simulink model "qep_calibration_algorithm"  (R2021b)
settings: Solver=FixedStepDiscrete  StartTime=0.0  StopTime=10.0  RelTol=1e-3
InitFcn:
  | qep_calibration_data;
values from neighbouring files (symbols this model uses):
  PWM_frequency = 20e3    (= 20000)    [qep_calibration_data.m]    (also in foc_qep_data.m; open_loop_data.m)
  Ts = 1/PWM_frequency    (= 5e-05)    [qep_calibration_data.m]    (also in foc_qep_data.m; open_loop_data.m)
undefined symbols (not defined in the file or in its folder): bits, motor
libraries: mcbcontrolslib x4, simulink x2, mcbpositiondecoderlib x2

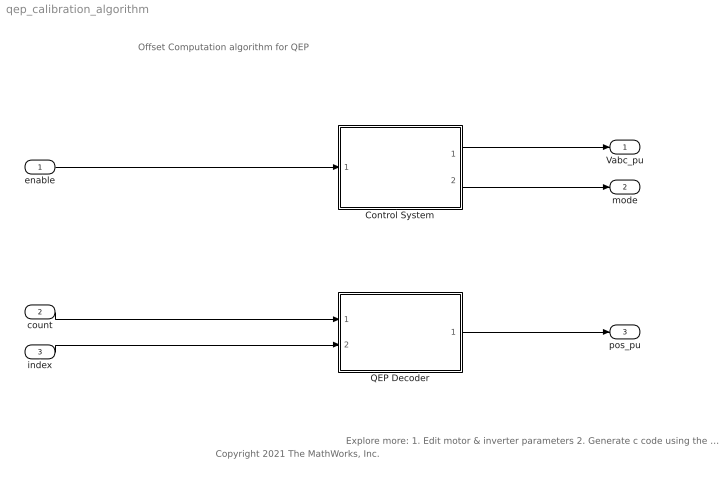
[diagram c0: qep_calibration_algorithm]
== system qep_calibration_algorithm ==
  note: Offset Computation algorithm for QEP
  note: Explore more: 1. Edit motor & inverter parameters 2. Generate c code using the 'Embedded Coder' app 3. Integrate generated code with driver code 4. Control motor via host model
  note: Copyright 2021 The MathWorks, Inc.
  enable : Inport  OutDataTypeStr=boolean
  count : Inport  Port=2  OutDataTypeStr=uint16
  index : Inport  Port=3  OutDataTypeStr=uint16
  Control System : Subsystem
  QEP Decoder : Subsystem
  Vabc_pu : Outport  OutDataTypeStr=dataType  VectorParamsAs1DForOutWhenUnconnected=off
  mode : Outport  Port=2  OutDataTypeStr=dataType
  pos_pu : Outport  Port=3  OutDataTypeStr=dataType
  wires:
  enable/1 -> Control System/1(Enable)
  Control System/1(Vabc_pu) -> Vabc_pu/1
  Control System/2(mode) -> mode/1
  count/1 -> QEP Decoder/1(Count)
  index/1 -> QEP Decoder/2(IndexCount)
  QEP Decoder/1(ϴe) -> pos_pu/1

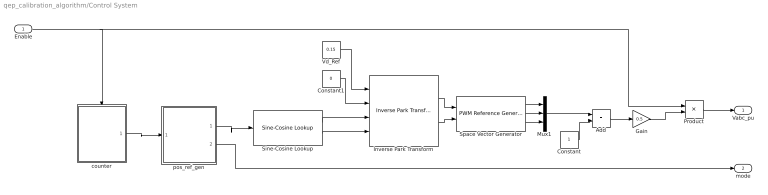
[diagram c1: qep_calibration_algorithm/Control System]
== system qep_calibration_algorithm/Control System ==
  Enable : Inport
  Add : Sum
  Constant : Constant  OutDataTypeStr=dataType
  Constant1 : Constant  Value=0  OutDataTypeStr=dataType  SampleTime=-1
  Gain : Gain  Gain=0.5
  Inverse Park Transform : mcbcontrolslib/Inverse Park Transform  AxisAlignment=D-axis
  Mux1 : Mux  Inputs=3
  Product : Product  OutDataTypeStr=dataType
  Sine-Cosine Lookup : mcbcontrolslib/Sine-Cosine Lookup  AngleInput=Per-unit  N_points=1024
  Space Vector Generator : mcbcontrolslib/PWM Reference Generator  inSignal=Valphabeta  modType=SVM: space vector modulation
  Vd_Ref : Constant  Value=0.15  OutDataTypeStr=dataType  SampleTime=-1
  counter : Subsystem
  pos_ref_gen : Subsystem
  Vabc_pu : Outport
  mode : Outport  Port=2
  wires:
  Sine-Cosine Lookup/2 -> Inverse Park Transform/4
  Inverse Park Transform/2 -> Space Vector Generator/2
  counter/1(count) -> pos_ref_gen/1(count)
  Space Vector Generator/3 -> Mux1/3
  Enable/1 -> counter/Enable, Product/1
  Vd_Ref/1 -> Inverse Park Transform/1
  Constant1/1 -> Inverse Park Transform/2
  Product/1 -> Vabc_pu/1
  Mux1/1 -> Add/1
  pos_ref_gen/1(pos_ref) -> Sine-Cosine Lookup/1
  Sine-Cosine Lookup/1 -> Inverse Park Transform/3
  Space Vector Generator/2 -> Mux1/2
  Inverse Park Transform/1 -> Space Vector Generator/1
  Gain/1 -> Product/2
  Space Vector Generator/1 -> Mux1/1
  pos_ref_gen/2(mode) -> mode/1
  Constant/1 -> Add/2
  Add/1 -> Gain/1

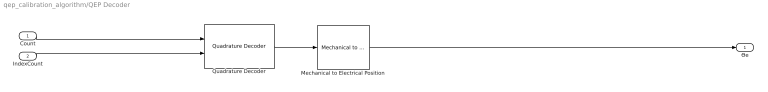
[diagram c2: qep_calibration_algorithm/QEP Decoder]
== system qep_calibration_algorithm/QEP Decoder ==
  Count : Inport
  IndexCount : Inport  Port=2
  Mechanical to Electrical Position : mcbpositiondecoderlib/Mechanical to Electrical Position  NrPP=motor.polepairs  selectedRange=Per unit  MechOfstInputType=Specify via dialog  mechOffsetIn=0  maxAngleIn=1  InputDataType=dataType  VariantSelect=floating-point
  Quadrature Decoder : mcbpositiondecoderlib/Quadrature Decoder  EncoderSlitsPerRevolution=motor.QEPSlits  EncoderCountsPerSlit=4  CounterSize=16 bits  ExternalIndexCount=on  PositionUnit=Per unit  PositionDataType=dataType
  ϴe : Outport
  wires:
  IndexCount/1 -> Quadrature Decoder/2
  Mechanical to Electrical Position/1 -> ϴe/1
  Quadrature Decoder/1 -> Mechanical to Electrical Position/1
  Count/1 -> Quadrature Decoder/1

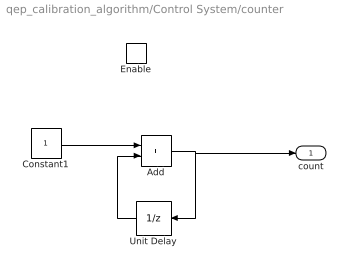
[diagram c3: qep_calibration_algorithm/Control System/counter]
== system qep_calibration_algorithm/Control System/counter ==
  Enable : EnablePort  StatesWhenEnabling=reset
  Add : Sum
  Constant1 : Constant  OutDataTypeStr=uint32
  Unit Delay : UnitDelay  SampleTime=-1  HasFrameUpgradeWarning=on
  count : Outport  InitialOutput=0
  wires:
  Unit Delay/1 -> Add/2
  Constant1/1 -> Add/1
  Add/1 -> count/1, Unit Delay/1

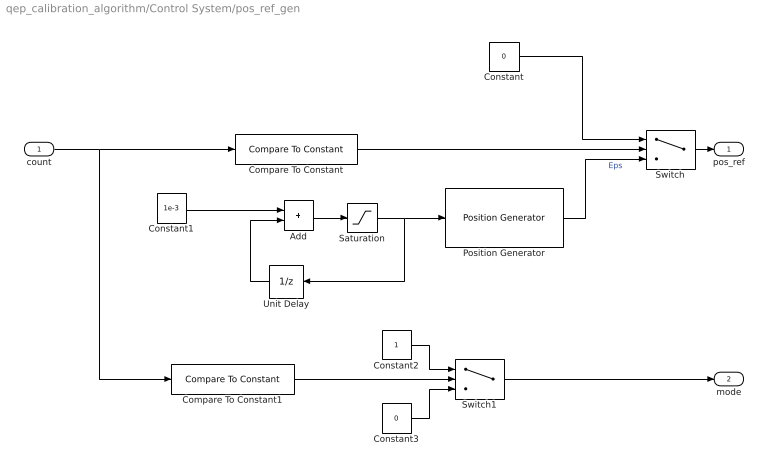
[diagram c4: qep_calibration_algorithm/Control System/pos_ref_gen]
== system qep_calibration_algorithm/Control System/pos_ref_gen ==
  count : Inport
  Add : Sum  OutDataTypeStr=single
  Compare To Constant : simulink/Logic and Bit Operations/Compare To Constant  relop=>=  const=10 * PWM_frequency  OutDataTypeStr=boolean
  Compare To Constant1 : simulink/Logic and Bit Operations/Compare To Constant  relop=>=  const=15 * PWM_frequency  OutDataTypeStr=boolean
  Constant : Constant  Value=0  OutDataTypeStr=dataType
  Constant1 : Constant  Value=1e-3  OutDataTypeStr=dataType
  Constant2 : Constant  OutDataTypeStr=dataType
  Constant3 : Constant  Value=0  OutDataTypeStr=dataType
  Position Generator : mcbcontrolslib/Position Generator  AngleOutput=Per-unit  ThetaSource=External  ThetaInput=5e-4  DataType=double  ExternalReset=none
  Saturation : Saturate  UpperLimit=motor.polepairs * Ts
  Switch : Switch  Criteria=u2 > Threshold
  Switch1 : Switch  Criteria=u2 > Threshold
  Unit Delay : UnitDelay  SampleTime=-1  HasFrameUpgradeWarning=on
  pos_ref : Outport
  mode : Outport  Port=2
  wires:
  Position Generator/1 -> Switch/3  "Eps"
  Constant/1 -> Switch/1
  Switch/1 -> pos_ref/1
  Add/1 -> Saturation/1
  Compare To Constant/1 -> Switch/2
  Unit Delay/1 -> Add/2
  Constant1/1 -> Add/1
  count/1 -> Compare To Constant1/1, Compare To Constant/1
  Compare To Constant1/1 -> Switch1/2
  Constant2/1 -> Switch1/1
  Constant3/1 -> Switch1/3
  Switch1/1 -> mode/1
  Saturation/1 -> Position Generator/1, Unit Delay/1
